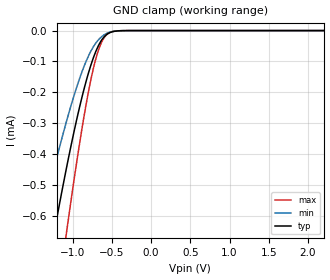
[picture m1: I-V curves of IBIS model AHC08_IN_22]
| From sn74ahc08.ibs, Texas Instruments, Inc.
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[Model]   AHC08_IN_22
Model_type  Input
Vinl = 0.5
Vinh = 1.56
| variable   typ   min   max
C_comp   0.83pF   0.76pF   0.91pF
[Temperature Range]   40   100   -40
| Ambient temperature   25   85   -40
[Voltage range]   2.2   2   2.4
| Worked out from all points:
|   GND clamp passes 1 mA (typ) near -1.47 V on its own axis
[GND Clamp]
| AHC08_IN_22
|   Voltage   I(typ)   I(min)   I(max)
-5.5V     -8.894mA   -6.578mA   -10.58mA
-1.465V   -992.3uA   -691.2uA   -1.41mA
-1.415V   -916.4uA   -636uA     -1.309mA
-1.265V   -697.1uA   -476.5uA   -1.01mA
-1.22V    -634.1uA   -430.8uA   -922.4uA
-1.08V    -447.6uA   -296.2uA   -658.7uA
-880mV    -215.2uA   -133.3uA   -316.8uA
-755mV    -102.6uA   -61.09uA   -144.8uA
-645mV    -36.78uA   -23.23uA   -46.24uA
-545mV    -9.057uA   -6.833uA   -9.231uA
-370mV    -356nA     -277.5nA   -177.8nA
2.2V      349.9pA    134.5pA    620.4pA
